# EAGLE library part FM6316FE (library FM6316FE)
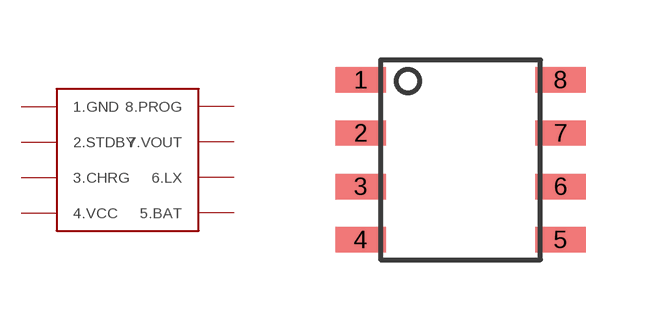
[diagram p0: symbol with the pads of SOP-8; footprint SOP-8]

Designator prefix -

## FM6316FE  [SOP-8]
1  1.GND
2  2.STDBY
3  3.CHRG
4  4.VCC
5  5.BAT
6  6.LX
7  7.VOUT
8  8.PROG

## Footprint SOP-8 (pad centres in mm)
smd 1.27 x 0.635: 1 -2.5,2; 2 -2.5,0.67; 3 -2.5,-0.67; 4 -2.5,-2; 5 2.5,-2; 6 2.5,-0.67; 7 2.5,0.67; 8 2.5,2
